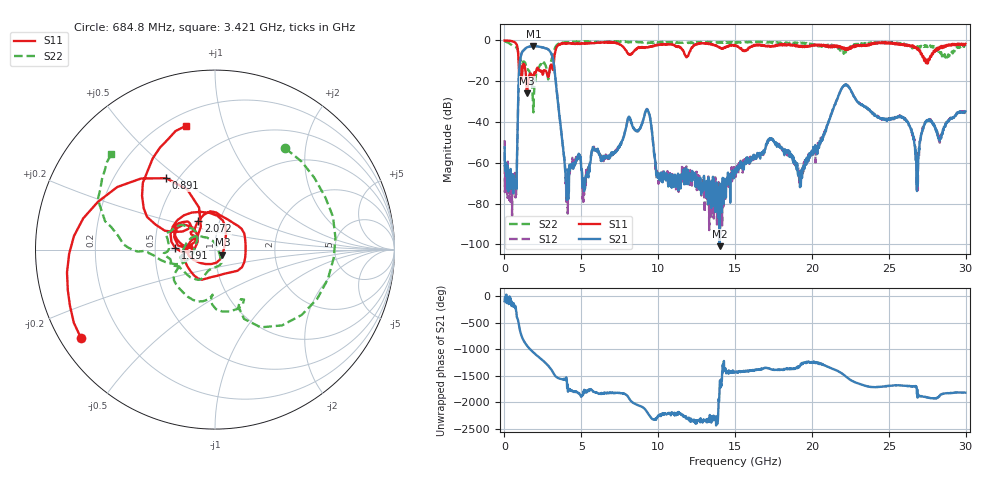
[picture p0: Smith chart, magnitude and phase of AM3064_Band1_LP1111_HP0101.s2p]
# Hz S DB R 50.0
!freq dBS11 angS11 dBS21 angS21 dBS12 angS12 dBS22 angS22
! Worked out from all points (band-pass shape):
!   1600 points, 10 MHz to 29.98 GHz, reference 50 ohm
!   highest |S21| = -2.73 dB at 1.884 GHz (marker M1); lowest = -100.9 dB at 13.99 GHz (marker M2)
!   |S21| within 3 dB of the highest: 1.153 GHz to 2.992 GHz (1.839 GHz wide, 88.7 % of centre)
!   lowest |S11| = -26.0 dB at 1.472 GHz (marker M3), VSWR 1.11, Z = 54.2 - j3.08 ohm
!   |S11| at or under -10 dB: 917.3 MHz to 3.221 GHz (2.304 GHz wide, 111 % of centre); 27.39266 GHz to 27.4592 GHz (66.54 MHz wide, 0.243 % of centre); 27.48885 GHz to 27.56356 GHz (74.7 MHz wide, 0.271 % of centre)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
!   |S22| runs from -35.3 to -0.2 dB; largest |S21 - S12| = 0.013
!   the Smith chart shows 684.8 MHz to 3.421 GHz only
!   S11 on the Smith chart (normalised r, x): 684.8 MHz: 0.06, -0.30; 891 MHz: 0.43, +0.45; 1.191 GHz: 0.64, +0.01; 2.072 GHz: 0.79, +0.26; 3.421 GHz: 0.27, +0.75
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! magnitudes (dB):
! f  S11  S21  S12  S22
! 10 MHz  0.0  -52.4  -49.0  -0.2
! 684.8 MHz  -1.0  -72.4  -65.0  -3.3
! 891 MHz  -6.3  -30.0  -29.9  -6.0
! 1.191 GHz  -13.1  -5.3  -5.3  -11.0
! 1.472 GHz  -26.0  -3.4  -3.3  -14.2
! 1.884 GHz  -17.7  -2.7  -2.8  -35.3
! 2.072 GHz  -14.7  -2.9  -2.8  -15.7
! 3.028 GHz  -11.9  -6.2  -6.1  -10.2
! 3.421 GHz  -3.0  -26.5  -26.3  -2.1
! 4.04 GHz  -1.5  -76.7  -71.9  -0.9
! 5.015 GHz  -1.6  -63.6  -62.8  -0.5
! 9.269 GHz  -3.4  -33.8  -33.6  -1.2
! 10 GHz  -2.2  -65.2  -67.0  -0.9
! 13.99 GHz  -3.3  -100.9  -75.2  -0.9
! 15 GHz  -2.6  -64.0  -65.3  -1.3
! 19.99 GHz  -2.8  -54.7  -55.3  -1.7
! 22.13 GHz  -4.3  -22.1  -22.0  -5.3
! 25 GHz  -1.0  -38.5  -38.4  -1.0
! 26.21 GHz  -2.2  -39.9  -40.1  -2.8
! 26.83 GHz  -4.2  -73.9  -64.8  -3.3
! 27.49 GHz  -10.0  -39.5  -39.1  -3.0
! 29.98 GHz  -1.7  -34.9  -35.0  -2.8
